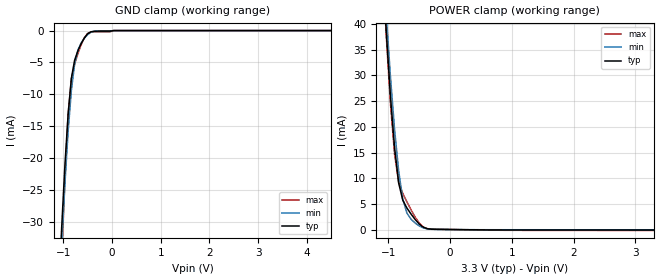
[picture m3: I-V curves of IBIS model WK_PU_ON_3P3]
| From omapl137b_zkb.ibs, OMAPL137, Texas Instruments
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|   Model Cell WK_PU_ON_3P3
|WK_PU_ON_3P3
[Model]   WK_PU_ON_3P3
Model_type   Input
Polarity   Non-Inverting
Vinl =  0.8
Vinh =  2
C_comp   1.652921p   1.424215p   1.79759p
[Model Spec]
Vinl   0.8   0.8   0.8
Vinh   2   2   2
[Temperature Range]   25   125   -40
[Voltage Range]   3.3   2.97   3.63
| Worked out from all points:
|   GND clamp passes 1 mA (typ) near -0.55 V on its own axis
|   POWER clamp passes 1 mA (typ) near -0.49 V on its own axis
| Nom Voltages:
|   VDD=1, VDDS=3.3, VSS=0, VSSS=0
| Min Voltages:
|   VDD=0.99, VDDS=2.97, VSS=0, VSSS=0
| Max Voltages:
|   VDD=1.21, VDDS=3.63, VSS=0, VSSS=0
[POWER_clamp]
|   voltage   I(typ)   I(min)   I(max)
-3.3V     637.1mA    797mA      659.4mA
-1.1V     52.51mA    55.16mA    52.59mA
-1.033V   38.38mA    41.76mA    37.53mA
-966.7mV  26.01mA    29.81mA    24.55mA
-900mV    16.01mA    19.59mA    14.66mA
-833.3mV  9.071mA    11.44mA    9.214mA
-766.7mV  5.724mA    5.931mA    7.03mA
-700mV    4.202mA    3.224mA    5.401mA
-500mV    1.081mA    706.3uA    1.257mA
-433.3mV  450.5uA    318.7uA    470.6uA
-300mV    74.15uA    53.23uA    103.8uA
3.3V      -90.11uA   -70.68uA   -183.1uA
[GND_clamp]
|   voltage   I(typ)   I(min)   I(max)
-3.3V     -540.4mA   -632.1mA   -650.2mA
-1.1V     -42.24mA   -44.8mA    -50.48mA
-1.033V   -30.98mA   -33.93mA   -36.16mA
-966.7mV  -21.17mA   -24.12mA   -23.24mA
-900mV    -13.09mA   -15.78mA   -13.05mA
-833.3mV  -7.473mA   -9.363mA   -7.573mA
-766.7mV  -4.639mA   -5.212mA   -5.254mA
-700mV    -3.171mA   -3.065mA   -3.635mA
-566.7mV  -1.148mA   -1.189mA   -1.104mA
-433.3mV  -198.7uA   -270.9uA   -234.1uA
33.33mV   0A         0A         0A
6.6V      0A         0A         0A
